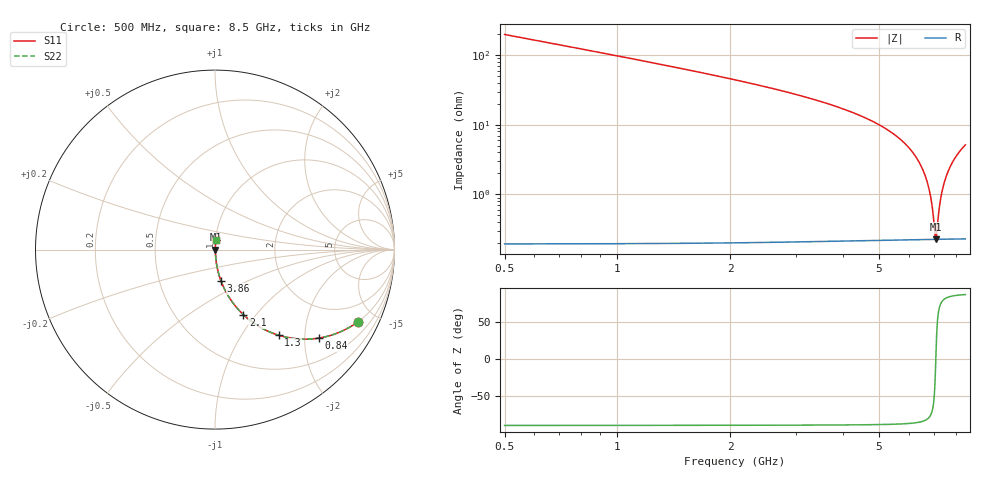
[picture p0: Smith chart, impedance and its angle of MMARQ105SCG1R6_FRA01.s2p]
! MMARQ105SCG1R6_FRA01  S-PARAMETER MODEL  ( General Type )
! Model Generated by TAIYO YUDEN Corporation (http://www.ty-top.com)
! Version 1.0
! TAIYO YUDEN Control No. 200326
! Copyright(c) 2020 TAIYO YUDEN CO.,LTD. All Rights Reserved.
! Product Description (link to TY-COMPAS)
! https://ds.yuden.co.jp/TYCOMPAS/or/detail?pn=MMARQ105SCG1R6BFRA01&u=M
! Products Name : Multilayer Ceramic Capacitors
! Characteristics :
!  Capacitance : 1.6 pF , Rated Voltage : 250V , TCC : CG / C0G
!  Case Size : 1.0 x 0.5 / 0.039 x 0.02 [mm/inch] , Thickness : 0.5 / 0.02 [mm/inch]
!  (Conditions: Temperature = 25 degC , DC Bias Current/Voltage = 0A / 0V)
! External Node Assignments :
!  1  o---| |---o  2
! GND o---------o GND
! Frequency Range : 500MHz  -  8.5GHz  [ 401 STEP ]
# MHz S RI R 50
! Freq[MHz].  S11 Real  S11 Imag  S21 Real  S21 Imag  S12 Real  S12 Imag  S22 Real  S22 Imag
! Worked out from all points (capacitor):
!   401 points, 500 MHz to 8.5 GHz, reference 50 ohm
!   read as one part in series: C = 1.6 pF near 540 MHz
!   lowest |Z| = 227 mohm at 7.08 GHz (marker M1)
!   series resonance near 7.086 GHz, so ESL is about 320 pH
!   S11 on the Smith chart (normalised r, x): 500 MHz: 1.00, -3.96; 840 MHz: 1.00, -2.34; 1.3 GHz: 1.00, -1.48; 2.1 GHz: 1.00, -0.86; 3.86 GHz: 1.00, -0.36; 8.5 GHz: 1.00, +0.10
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500  0.7968 -0.4019  0.2032 0.4019  0.2032 0.4019  0.7968 -0.4019
840  0.5772 -0.4932  0.4228 0.4932  0.4228 0.4932  0.5772 -0.4932
1300  0.3543 -0.477  0.6457 0.477  0.6457 0.477  0.3543 -0.477
1840  0.2039 -0.4009  0.7961 0.4009  0.7961 0.4009  0.2039 -0.4009
2100  0.1587 -0.3631  0.8413 0.3631  0.8413 0.3631  0.1587 -0.3631
3180  0.0605 -0.2343  0.9395 0.2343  0.9395 0.2343  0.0605 -0.2343
3860  0.0337 -0.1748  0.9663 0.1748  0.9663 0.1748  0.0337 -0.1748
4500  0.0192 -0.1291  0.9808 0.1291  0.9808 0.1291  0.0192 -0.1291
5840  0.00517 -0.0543  0.9948 0.0543  0.9948 0.0543  0.00517 -0.0543
6340  0.0032 -0.0311  0.9968 0.0311  0.9968 0.0311  0.0032 -0.0311
6680  0.00251 -0.0165  0.9975 0.0165  0.9975 0.0165  0.00251 -0.0165
6880  0.00232 -0.00826  0.9977 0.00826  0.9977 0.00826  0.00232 -0.00826
6960  0.00227 -0.00503  0.9977 0.00503  0.9977 0.00503  0.00227 -0.00503
7040  0.00226 -0.00184  0.9977 0.00184  0.9977 0.00184  0.00226 -0.00184
7080  0.00225 -0.000255  0.9977 0.000255  0.9977 0.000255  0.00225 -0.000255
7120  0.00226 0.00132  0.9977 -0.00132  0.9977 -0.00132  0.00226 0.00132
7180  0.00227 0.00366  0.9977 -0.00366  0.9977 -0.00366  0.00227 0.00366
7260  0.0023 0.00676  0.9977 -0.00676  0.9977 -0.00676  0.0023 0.00676
7340  0.00236 0.00982  0.9976 -0.00982  0.9976 -0.00982  0.00236 0.00982
7600  0.00265 0.0196  0.9974 -0.0196  0.9974 -0.0196  0.00265 0.0196
7980  0.00338 0.0332  0.9966 -0.0332  0.9966 -0.0332  0.00338 0.0332
8500  0.0049 0.051  0.9951 -0.051  0.9951 -0.051  0.0049 0.051
